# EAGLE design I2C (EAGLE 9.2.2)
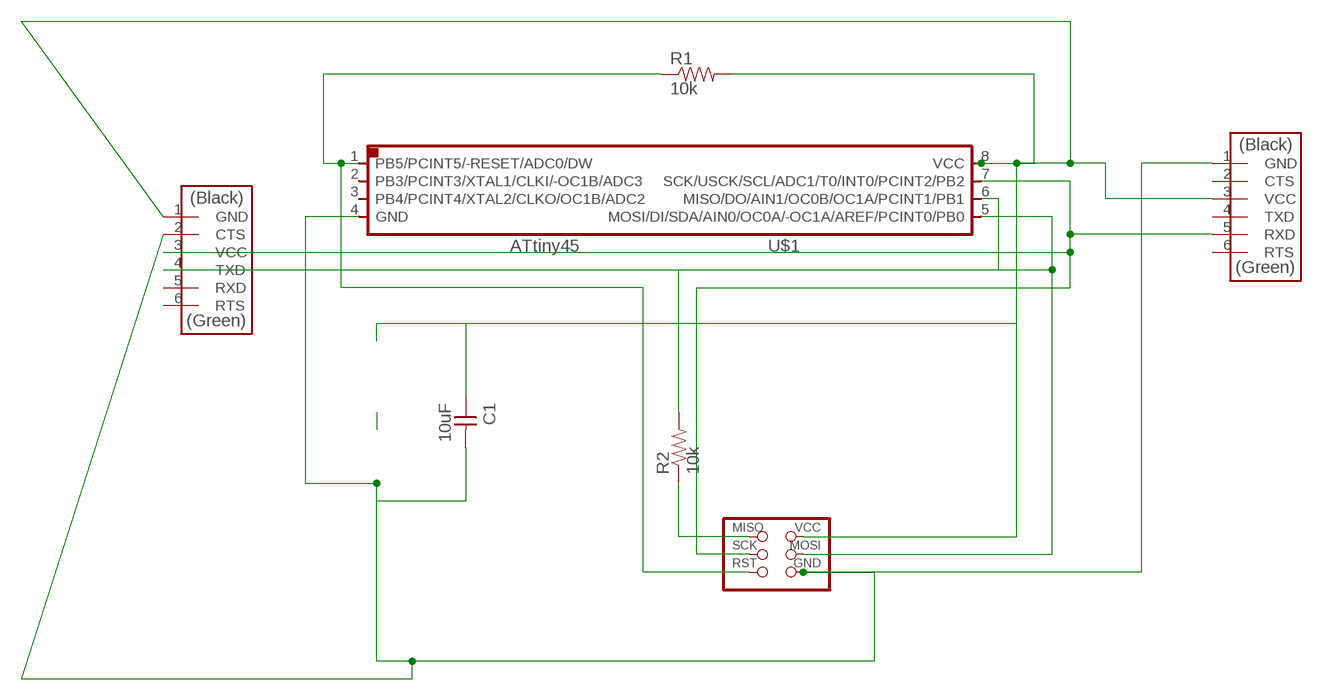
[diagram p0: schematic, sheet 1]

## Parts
C1  10uF  CAP-UNPOLARIZEDFAB  [C1206FAB]
FTDI  FTDI-SMD-HEADER  [1X06SMD]
FTDI1  FTDI-SMD-HEADER  [1X06SMD]
ISP  AVRISPSMD  [2X03SMD]
R1  10k  RESISTOR1206  [1206]
R2  10k  RESISTOR1206  [1206]
U$1  ATTINY45SI  [SOIC8]

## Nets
N$2: ISP.1(MISO) R2.1
N$3: C1.2 FTDI1.2(CTS) FTDI.1(GND) ISP.6(GND) U$1.4(GND)
N$4: ISP.5(RST) R1.1 U$1.1(PB5/PCINT5/-RESET/ADC0/DW)
N$5: FTDI1.3(VCC) FTDI.5(RXD) ISP.3(SCK) U$1.7(SCK/USCK/SCL/ADC1/T0/INT0/PCINT2/PB2)
N$7: FTDI1.4(TXD) ISP.4(MOSI) U$1.5(MOSI/DI/SDA/AIN0/OC0A/-OC1A/AREF/PCINT0/PB0)
N$8: R2.2 U$1.6(MISO/DO/AIN1/OC0B/OC1A/PCINT1/PB1)
N$9: C1.1 FTDI1.1(GND) FTDI.3(VCC) ISP.2(VCC) R1.2 U$1.8(VCC)
Unconnected: FTDI1.5(RXD) FTDI1.6(RTS) FTDI.2(CTS) FTDI.4(TXD) FTDI.6(RTS) U$1.2(PB3/PCINT3/XTAL1/CLKI/-OC1B/ADC3) U$1.3(PB4/PCINT4/XTAL2/CLKO/OC1B/ADC2)

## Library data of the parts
C1 = fab:CAP-UNPOLARIZED
FTDI FTDI1 = fab:FTDI-SMD-HEADER
ISP = fab:AVRISP
R1 R2 = SparkFun-Resistors:RESISTOR: Generic Resistor Package
U$1 = fab:ATTINY45

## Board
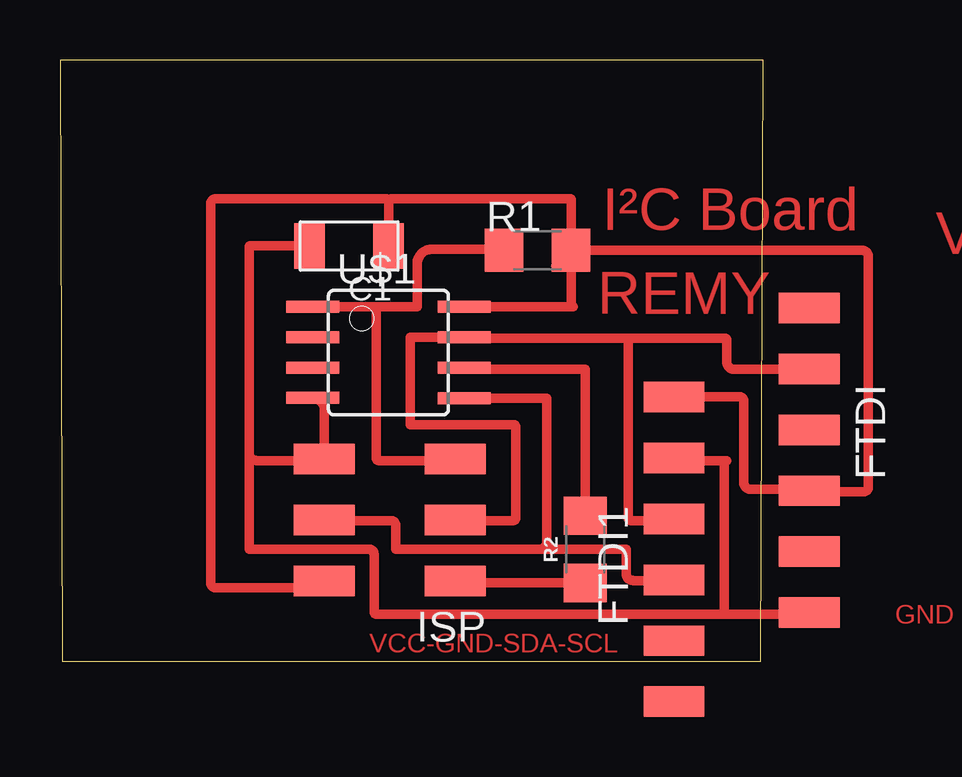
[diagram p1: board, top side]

Size 29.3 x 25.06 mm. Coordinates in mm from the lower left corner, seen from the top.
Outline: 0.1,0 29.2,0 29.3,25.06 0,25.06 0.1,0
Copper layers (1*16): Top 0.035mm / dielectric 1.5mm / Bottom 0.035mm
Design rules "default *": minimum track width 0.4mm, minimum drill 0.4mm, track to track 0.3mm, track to pad 0.3mm, pad to pad 0.3mm, via to via 6mil, smd to smd 0.3mm, copper to edge 40mil, drill to drill 6mil, minimum pad ring 10mil, minimum via ring 8mil, stop-mask expansion 4mil, vias tented up to drill 0mil, thermal gap 10mil

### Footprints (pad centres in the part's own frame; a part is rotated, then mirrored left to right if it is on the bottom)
C1206FAB = smd 1.27 x 1.905: 1 -1.651,0; 2 1.651,0
1X06SMD = smd 2.54 x 1.27: 1 0,6.35; 2 0,3.81; 3 0,1.27; 4 0,-1.27; 5 0,-3.81; 6 0,-6.35
2X03SMD = smd 2.54 x 1.27: 1 -2.54,2.54; 2 2.92,2.54; 3 -2.54,0; 4 2.92,0; 5 -2.54,-2.54; 6 2.92,-2.54
1206 = smd 1.6 x 1.8: 1 -1.4,0; 2 1.4,0
SOIC8 = smd 0.5 x 2.2: 1 -1.905,-3.154; 2 -0.645,-3.154; 3 0.625,-3.154; 4 1.895,-3.154; 5 1.905,3.154; 6 0.635,3.154; 7 -0.635,3.154; 8 -1.905,3.154

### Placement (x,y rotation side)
C1  12.04,17.31 180 top
FTDI  31.22,8.38 180 top
FTDI1  25.58,4.67 0 top
ISP  13.93,5.89 180 top
R1  19.89,17.13 0 top
R2  21.88,4.67 90 top
U$1  13.68,12.87 270 top

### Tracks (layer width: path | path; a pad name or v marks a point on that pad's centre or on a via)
N$2
  Top 0.4: ISP.1 arc-90 16.48,3.34 | ISP.1 arc-90 16.49,3.37 | ISP.1 arc90 16.55,3.27 R2.1
N$3
  Top 0.4: U$1.4 arc-90 11.01,10.5 ISP.6 | ISP.6 arc-90 10.95,8.37 8.18,8.37 arc-90 7.88,8.67 | 7.88,8.67 7.88,17.27 arc-90 7.92,17.31 C1.2 | ISP.6 arc90 10.88,8.31 | 7.88,8.67 7.88,4.67 12.88,4.67 arc-90 13.08,4.47 13.08,2.07 arc90 13.18,1.97 27.68,1.97 | 31.16,1.97 arc90 FTDI.1 arc-90 31.16,1.97 | 25.67,8.57 arc90 FTDI1.2 arc90 25.69,8.37 27.78,8.37 arc90 27.68,8.27 27.68,1.97 | 31.16,1.97 27.68,1.97
N$4
  Top 0.4: ISP.5 arc-90 16.41,8.37 13.28,8.37 arc-90 13.18,8.47 13.18,14.77 arc90 13.18,14.78 | 13.18,14.78 10.78,14.78 U$1.1 | R1.1 arc90 18.45,17.17 15.48,17.17 arc90 14.88,16.57 14.88,14.77 arc90 14.88,14.78 13.18,14.78
N$5
  Top 0.4: ISP.3 arc90 16.49,5.87 18.88,5.87 arc90 18.98,5.97 18.98,9.77 arc90 18.88,9.87 14.58,9.87 14.58,13.47 arc-90 14.62,13.51 U$1.7 arc90 16.87,13.47 23.68,13.47 | FTDI.5 arc-90 31.2,12.17 28.08,12.17 arc-90 27.78,12.47 27.78,13.37 arc90 27.68,13.47 23.68,13.47 | FTDI1.3 arc-90 25.51,5.87 23.78,5.87 arc-90 23.68,5.97 23.68,13.47
N$7
  Top 0.4: 11.13,5.77 arc-90 ISP.4 arc90 11.03,5.87 13.78,5.87 arc-90 13.98,5.67 13.98,4.67 19.68,4.67 19.98,4.67 | 19.98,4.67 arc90 20.28,4.97 20.28,10.97 arc-90 20.28,10.97 U$1.5 | FTDI1.4 arc-90 25.55,3.37 23.88,3.37 arc-90 23.58,3.67 23.58,4.67 19.98,4.67
N$8
  Top 0.4: 16.87,12.27 arc90 U$1.6 arc90 16.9,12.17 21.88,12.17 R2.2
N$9
  Top 0.4: R1.2 20.66,16.49 | FTDI.3 arc-90 31.28,7.17 | ISP.2 arc-90 10.73,3.07 6.48,3.07 arc-90 6.28,3.27 6.28,19.07 arc-90 6.48,19.27 13.58,19.27 arc-90 13.7,19.16 | C1.1 13.7,19.16 | R1.2 21.29,19.26 arc90 21.28,19.27 13.81,19.27 arc90 13.7,19.16 | U$1.8 arc90 U$1.8 21.38,14.77 arc-90 21.29,14.86 R1.2 | FTDI.3 arc90 31.16,7.17 28.78,7.17 arc-90 28.48,7.47 28.48,10.87 arc90 28.33,11.02 FTDI1.1 | FTDI.3 arc90 31.26,7.07 33.48,7.07 arc90 33.68,7.27 33.68,16.87 arc90 33.42,17.13 R1.2

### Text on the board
Top: I²C Board | VCC | REMY | GND | VCC-GND-SDA-SCL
